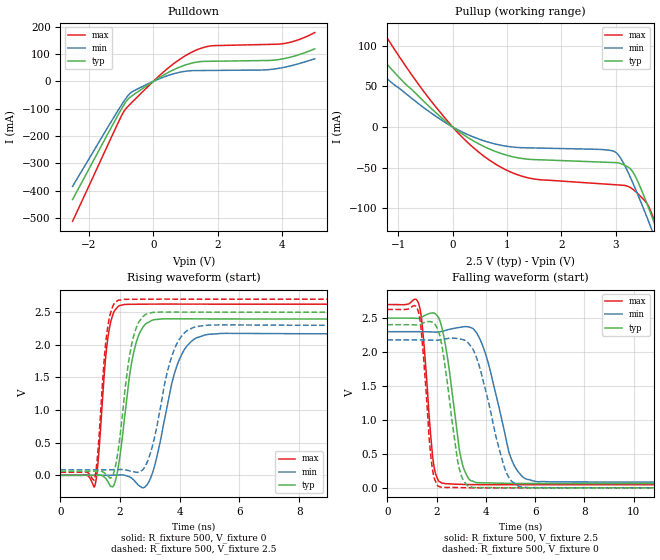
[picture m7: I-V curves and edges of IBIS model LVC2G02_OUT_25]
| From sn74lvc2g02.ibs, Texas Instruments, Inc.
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[Model]   LVC2G02_OUT_25
Model_type  Output
Vref =   0
Rref =   500
Cref =   30p
Vmeas =   1.25
| variable   typ   min   max
C_comp   9.09pF   6.56pF   15.51pF
| C_pullup   8.08pF   6.56pF   8.97pF
| C_pulldown   10.09pF   6.58pF   15.51pF
[Temperature Range]   40   100   -40
| Ambient temperature   25   85   -40
[Voltage range]   2.5   2.3   2.7
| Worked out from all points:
|   slope of the pulldown table from 0 to 0.375 V, typ, clamps not added: 13.9 ohm
|   slope of the pullup table from 0 to 0.375 V, typ, clamps not added: 22.2 ohm
|   rising waveform, R_fixture 500, V_fixture 0: 20-80 % time 426ps typ, 645ps min, 273ps max; typ from 0 V to 2.4 V
|   falling waveform, R_fixture 500, V_fixture 2.5: 20-80 % time 530ps typ, 851ps min, 335ps max; typ from 2.5 V to 0.063 V
|   rising waveform, R_fixture 500, V_fixture 2.5: 20-80 % time 406ps typ, 632ps min, 263ps max; typ from 0.063 V to 2.5 V
|   falling waveform, R_fixture 500, V_fixture 0: 20-80 % time 531ps typ, 874ps min, 322ps max; typ from 2.4 V to 0 V
[Pulldown]
| LVC2G02_OUT_25
|   Voltage   I(typ)   I(min)   I(max)
-2.5V     -431.9mA   -384.1mA   -511.5mA
-1.16V    -137.7mA   -119.4mA   -169.2mA
-900mV    -84.06mA   -71.1mA    -107.9mA
-780mV    -64.71mA   -51.71mA   -91.11mA
-615mV    -49.34mA   -35.5mA    -71.41mA
570mV     38.99mA    25.71mA    59.05mA
1.135V    64.89mA    38.7mA     103.2mA
1.645V    73.21mA    39.77mA    126.7mA
3.415V    76.06mA    41.68mA    134.7mA
4V        81.99mA    50.17mA    137.5mA
4.475V    96.16mA    63.62mA    151.2mA
5V        118.9mA    82.47mA    178.4mA
[Pullup]
| LVC2G02_OUT_25
|   Voltage   I(typ)   I(min)   I(max)
-2.5V     185.9mA    146.6mA    260.1mA
-2.08V    148.4mA    116.3mA    208.5mA
-1.78V    122.8mA    95.69mA    173.1mA
-1.315V   85.46mA    65.95mA    121.2mA
-45mV     2.35mA     1.738mA    3.424mA
965mV     -34.17mA   -23.43mA   -52.22mA
1.54V     -40.26mA   -25.92mA   -64.43mA
2.97V     -43.8mA    -30.07mA   -70.97mA
3.295V    -53.49mA   -65.76mA   -75.7mA
3.645V    -106.6mA   -123mA     -103.6mA
3.77V     -129.2mA   -144.6mA   -126.2mA
5V        -368.9mA   -369.6mA   -390mA
[Ramp]
| LVC2G02_OUT_25
| variable   typ   min   max
dV/dt_r   1.55/4.62E-10   1.42/7.16E-10   1.68/2.91E-10
dV/dt_f   1.51/5.62E-10   1.38/9.10E-10   1.64/3.54E-10
R_load = 500
[Rising Waveform]
| LVC2G02_OUT_25
R_fixture =   500
C_fixture =   0
L_fixture =   0
V_fixture =   0
V_fixture_min = 0
V_fixture_max = 0
|   Time   V(typ)   V(min)   V(max)
0s        178.4nV    -218.8nV   121.7nV
1.15ns    1.308mV    -63.91uV   -163.8mV
1.585ns   -91.86mV   -79.74uV   2.087V
1.795ns   -146.8mV   1.982mV    2.507V
2.005ns   331.3mV    5.107mV    2.606V
2.48ns    1.933V     -82.61mV   2.622V
3.145ns   2.386V     126.5mV    2.624V
3.95ns    2.398V     1.735V     2.625V
4.9ns     2.398V     2.157V     2.624V
24.99ns   2.396V     2.17V      2.624V
[Falling Waveform]
| LVC2G02_OUT_25
R_fixture =   500
C_fixture =   0
L_fixture =   0
V_fixture =   2.5
V_fixture_min = 2.3
V_fixture_max = 2.7
|   Time   V(typ)   V(min)   V(max)
0s        2.5V       2.3V       2.7V
1.285ns   2.497V     2.3V       2.7V
1.47ns    2.528V     2.3V       2.189V
1.86ns    2.576V     2.296V     402.9mV
2.23ns    2.339V     2.306V     67.59mV
2.995ns   432.5mV    2.367V     51.13mV
3.59ns    78.77mV    2.3V       47.07mV
4.96ns    65.92mV    500.1mV    46.5mV
5.68ns    63.8mV     123.9mV    46.69mV
24.99ns   63.48mV    83.95mV    46.77mV
[Rising Waveform]
| LVC2G02_OUT_25
R_fixture =   500
C_fixture =   0
L_fixture =   0
V_fixture =   2.5
V_fixture_min = 2.3
V_fixture_max = 2.7
|   Time   V(typ)   V(min)   V(max)
0s        63.44mV    83.88mV    46.75mV
1.135ns   64.41mV    83.83mV    -66.34mV
1.56ns    3.574mV    83.75mV    2.193V
1.965ns   484.9mV    88.43mV    2.687V
2.32ns    1.843V     66.7mV     2.698V
2.63ns    2.352V     49.78mV    2.699V
3.04ns    2.492V     377.6mV    2.7V
3.825ns   2.502V     1.94V      2.701V
4.58ns    2.501V     2.283V     2.7V
24.99ns   2.5V       2.3V       2.7V
[Falling Waveform]
| LVC2G02_OUT_25
R_fixture =   500
C_fixture =   0
L_fixture =   0
V_fixture =   0
V_fixture_min = 0
V_fixture_max = 0
|   Time   V(typ)   V(min)   V(max)
0s        2.403V     2.179V     2.628V
1.25ns    2.399V     2.179V     2.608V
1.395ns   2.414V     2.179V     2.25V
1.81ns    2.443V     2.175V     335.9mV
2.2ns     2.125V     2.183V     6.779mV
2.86ns    386.3mV    2.199V     3.744mV
3.315ns   20.34mV    2.122V     873.7uV
4.78ns    1.254mV    271.7mV    -242.5uV
5.405ns   373.3nV    14.42mV    -66.27uV
24.99ns   36.39uV    58.29uV    24.1uV
